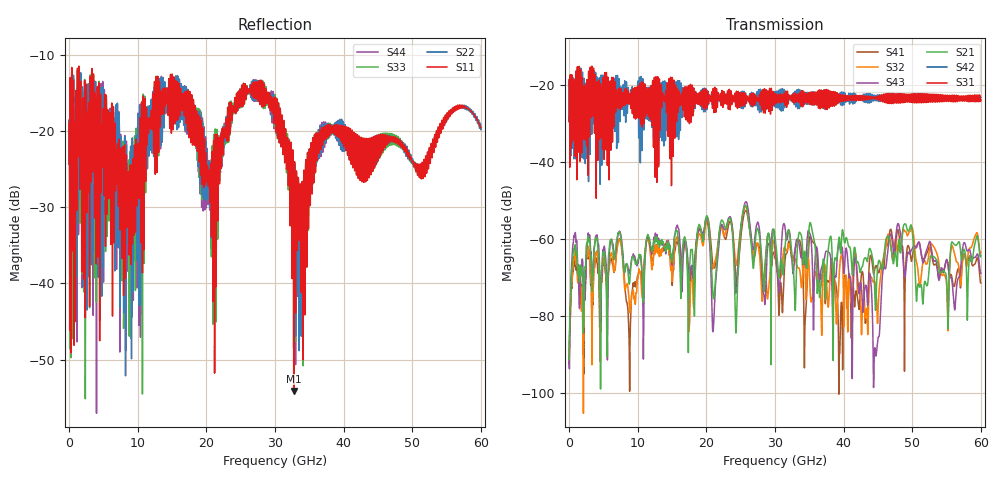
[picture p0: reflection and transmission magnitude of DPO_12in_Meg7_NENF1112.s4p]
! Tyco Electronics Strada Whisper System
! NEXT_F1112_G1112
!! SYSTEM DESCRIPTION: Daughtercard-Footprint-Connector-Footprint-Daughtercard
!! PCB DESCRIPTION: DC: 140mil, Megtron7N, upper layer route, 15mil stub, 6-6-6mil 12" traces
!! CONNECTOR DESCRIPTION: Next-Gen STRADA Whisper Direct-Plug Orthogonal Connector
!! MODEL DESCRIPTION: Tyco Electronics System 4-port S-parameter
!! MODEL STATUS: Developmental
!! MODEL GEOMETRY: Channel Model
!! MODEL FREQUENCY RANGE: DC to 60 GHz in 10 MHz frequency steps
!! MODEL EDGE RATE LIMITATION: 8.3 ps (Using conservative 0.5/Fmax rule of thumb)
!! TIME-DOMAIN TRANSFORM CAUTIONS:
!! 1.) Do not simulate transient edge rates faster than the number listed above.  Edge rates faster than this number
!!  contain significant spectral content at frequencies above the model's highest frequency.
!! 2.) Even when simulating edge rates that are slower than the number listed above, be aware that the best time
!!  resolution possible with a direct iFFT is (1 / 2Fmax).  As a result, time resolution is typically not adequate
!!  for most time-domain simulations unless tricks such as windowing are used to minimize leakage and aliasing.
!! 3.) Because the model has a uniform frequency step, a direct iFFT will result in an impulse that that has a time
!!  length given by either (1 / Fstep) or (1 / 2Fstep), depending on the transform being used.  Care has been taken
!!  in selecting the frequency step to ensure a settled impulse response for the model.  Therefore, convolution with
!!  the model's impulse response should present no issues.  However, if directly concatenating s-parameter models
!!  in the frequency domain a user must either interpolate necessary interim frequencies or complete impulse response
!!  zero-padding.  Impulse response zero-padding is more difficult, but more accurate.
!! PORT DEFINITIONS:
!! Port  1  ----->  RX Side	F11  G11  RX Side  <-----  Port  3
!! Port  2  ----->  RX Side	F12  G12  RX Side  <-----  Port  4
! Touchstone data
! Created: 10-Dec-2018 by IdEM R2012 (8.0.5)
# Hz S MA R 50
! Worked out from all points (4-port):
!   6000 points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, 10 MHz to 60 GHz, reference 50 ohm
!   strongest paths, dB at 10 MHz, 15.01 GHz, 30.01 GHz, 45.01 GHz, 60 GHz:
!     S31: -29.5, -18.6, -22.4, -23.1, -23.9
!     S42: -29.6, -25.0, -21.8, -23.0, -23.3
!     S21: -91.3, -66.0, -59.5, -66.6, -64.3
!     S43: -91.8, -66.8, -61.9, -85.8, -68.9
!     S32: -92.6, -71.0, -63.9, -79.4, -63.6
!     S41: -92.1, -71.7, -65.0, -68.5, -71.5
!   lowest |S11| = -54.1 dB at 32.73 GHz (marker M1), VSWR 1.00, Z = 50.2 + j0.105 ohm
!   |S11| at or under -10 dB: start of sweep to end of sweep
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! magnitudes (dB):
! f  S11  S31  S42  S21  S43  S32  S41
! 10 MHz  -24.2  -29.5  -29.6  -91.3  -91.8  -92.6  -92.1
! 20.07 GHz  -26.7  -23.9  -26.4  -54.0  -54.6  -55.5  -54.2
! 21 GHz  -30.0  -21.1  -21.6  -75.4  -83.7  -67.5  -67.1
! 24.36 GHz  -15.8  -22.3  -24.2  -82.9  -73.5  -66.8  -70.8
! 25.66 GHz  -13.8  -22.2  -23.6  -51.3  -50.5  -51.7  -52.7
! 32.73 GHz  -54.1  -24.0  -22.6  -69.3  -68.2  -65.3  -65.0
! 60 GHz  -19.6  -23.9  -23.3  -64.3  -68.9  -63.6  -71.5
